FUNCTION_BLOCK Example28a_zoneunloading //2x1 flyways 2 xbots (actual physical) - ZoneCtrl
VAR_INPUT
	Execute : BOOL;
	UserFinishedRemovingXbot : BOOL;
END_VAR
VAR_OUTPUT
	UserCanRemoveXbot : BOOL;
	Done : BOOL;
END_VAR
VAR_IN_OUT
	PM_Controller : PMControllerType;	// the planar motor controller to use
END_VAR
VAR
	xbotid_array78 : ARRAY[0..77] OF USINT;
	posx_array78 : ARRAY[0..77] OF REAL;
	posy_array78 : ARRAY[0..77] OF REAL;
	PMC_AutoDrivingMotion1 : PMC_AutoDrivingMotion;
	PMC_XYMotion1 : PMC_XYMotion;
	PMC_Zone_ZoneCtrl1 : PMC_Zone_ZoneCtrl;
	PMC_Zone_ZoneCtrl2 : PMC_Zone_ZoneCtrl;
END_VAR

//2x1 flyways 2 xbots (actual physical) - ZoneCtrl

IF NOT(Execute) THEN
	UserFinishedRemovingXbot := FALSE;
END_IF; 

//move to starting position
xbotid_array78[0] := 1; xbotid_array78[1] := 2;
posx_array78[0] := 0.06;posx_array78[1] := 0.18;
posy_array78[0] := 0.06;posy_array78[1] := 0.06;
PMC_AutoDrivingMotion1(Execute := Execute,nXbots := 2,RoutingType := 0,ZoneID := 0,XbotID := xbotid_array78,PosX := posx_array78,PosY := posy_array78,PM_Controller := PM_Controller);

//move xbot 2 into zone 2 (flyway 2)
PMC_XYMotion1(Execute := PMC_AutoDrivingMotion1.Done,cmdLB := 2,XbotID := 2,Mode := 0,Type_ := 0,PosX := 0.36,PosY := 0.12,EndVel := 0,MaxVel := 1,MaxAcc := 10,PM_Controller := PM_Controller);

//deactivate zone 2 (flyway 2)
PMC_Zone_ZoneCtrl1(Execute := PMC_XYMotion1.Done,ZoneID := 2,Level := 0,PM_Controller := PM_Controller);

//tell user that they can remove the xbot in the zone
UserCanRemoveXbot := PMC_Zone_ZoneCtrl1.Done;

//activate zone once user says they are done removing the xbot
PMC_Zone_ZoneCtrl2(Execute := UserFinishedRemovingXbot AND PMC_Zone_ZoneCtrl1.Done,ZoneID := 2,Level := 1,PM_Controller := PM_Controller);

Done := PMC_Zone_ZoneCtrl2.Done;

END_FUNCTION_BLOCK
